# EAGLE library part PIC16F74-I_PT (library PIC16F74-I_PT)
Microcontroller,PIC16F74-I/PT 20MHz PIC16F74-I/PT, 8 bit PIC Microcontroller 20MHz 4K x 14 words Flash, 192 B RAM, I2C 44-Pin TQFP Source: Datasheet
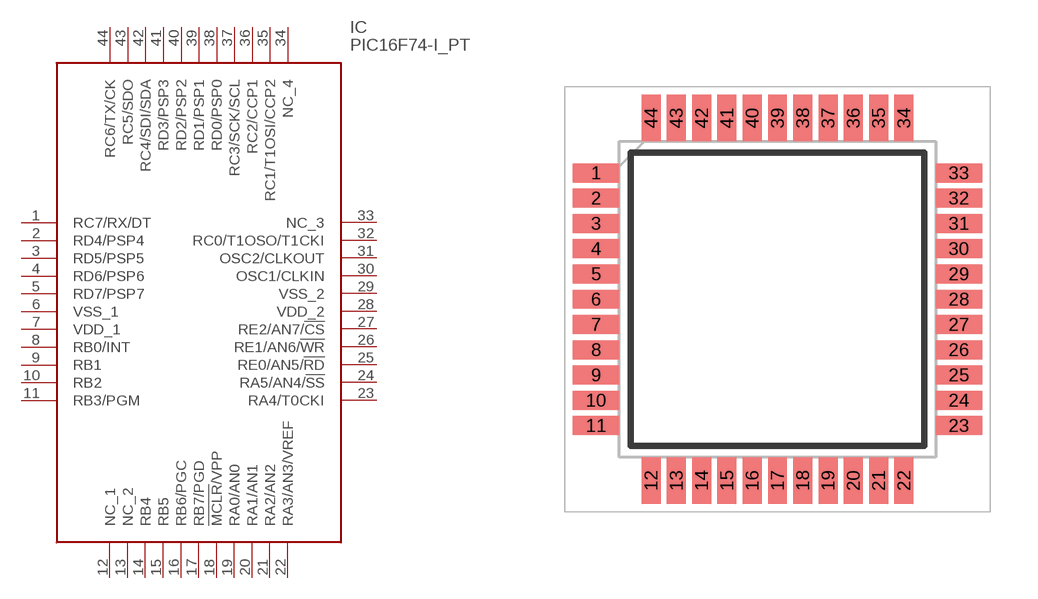
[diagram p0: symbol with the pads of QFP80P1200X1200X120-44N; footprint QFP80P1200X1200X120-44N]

Designator prefix IC

## PIC16F74-I_PT (Description: Microcontroller,PIC16F74-I/PT 20MHz PIC16F74-I/PT, 8 bit PIC Microcontroller 20MHz 4K x 14 words Flash, 192 B RAM, I2C 44-Pin TQFP; Height: 1.2mm; Manufacturer_Name: Microchip; Manufacturer_Part_Number: PIC16F74-I/PT; Mouser_Part_Number: 579-PIC16F74-I/PT; Mouser_Price-Stock: https://www.mouser.co.uk/ProductDetail/Microchip-Technology/PIC16F74-I-PT?qs=XNV0BZVlaZGqP4g9iwg2yA%3D%3D)  [QFP80P1200X1200X120-44N]
1  RC7/RX/DT
2  RD4/PSP4
3  RD5/PSP5
4  RD6/PSP6
5  RD7/PSP7
6  VSS_1
7  VDD_1
8  RB0/INT
9  RB1
10  RB2
11  RB3/PGM
12  NC_1
13  NC_2
14  RB4
15  RB5
16  RB6/PGC
17  RB7/PGD
18  !MCLR!/VPP
19  RA0/AN0
20  RA1/AN1
21  RA2/AN2
22  RA3/AN3/VREF
23  RA4/T0CKI
24  RA5/AN4/!SS
25  RE0/AN5/!RD
26  RE1/AN6/!WR
27  RE2/AN7/!CS
28  VDD_2
29  VSS_2
30  OSC1/CLKIN
31  OSC2/CLKOUT
32  RC0/T1OSO/T1CKI
33  NC_3
34  NC_4
35  RC1/T1OSI/CCP2
36  RC2/CCP1
37  RC3/SCK/SCL
38  RD0/PSP0
39  RD1/PSP1
40  RD2/PSP2
41  RD3/PSP3
42  RC4/SDI/SDA
43  RC5/SDO
44  RC6/TX/CK

## Footprint QFP80P1200X1200X120-44N (pad centres in mm)
(PT)44-Lead(TQFP)
smd 1.475 x 0.6: 1 -5.738,4; 2 -5.738,3.2; 3 -5.738,2.4; 4 -5.738,1.6; 5 -5.738,0.8; 6 -5.738,0; 7 -5.738,-0.8; 8 -5.738,-1.6; 9 -5.738,-2.4; 10 -5.738,-3.2; 11 -5.738,-4; 23 5.738,-4; 24 5.738,-3.2; 25 5.738,-2.4; 26 5.738,-1.6; 27 5.738,-0.8; 28 5.738,0; 29 5.738,0.8; 30 5.738,1.6; 31 5.738,2.4; 32 5.738,3.2; 33 5.738,4
smd 0.6 x 1.475: 12 -4,-5.738; 13 -3.2,-5.738; 14 -2.4,-5.738; 15 -1.6,-5.738; 16 -0.8,-5.738; 17 0,-5.738; 18 0.8,-5.738; 19 1.6,-5.738; 20 2.4,-5.738; 21 3.2,-5.738; 22 4,-5.738; 34 4,5.738; 35 3.2,5.738; 36 2.4,5.738; 37 1.6,5.738; 38 0.8,5.738; 39 0,5.738; 40 -0.8,5.738; 41 -1.6,5.738; 42 -2.4,5.738; 43 -3.2,5.738; 44 -4,5.738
